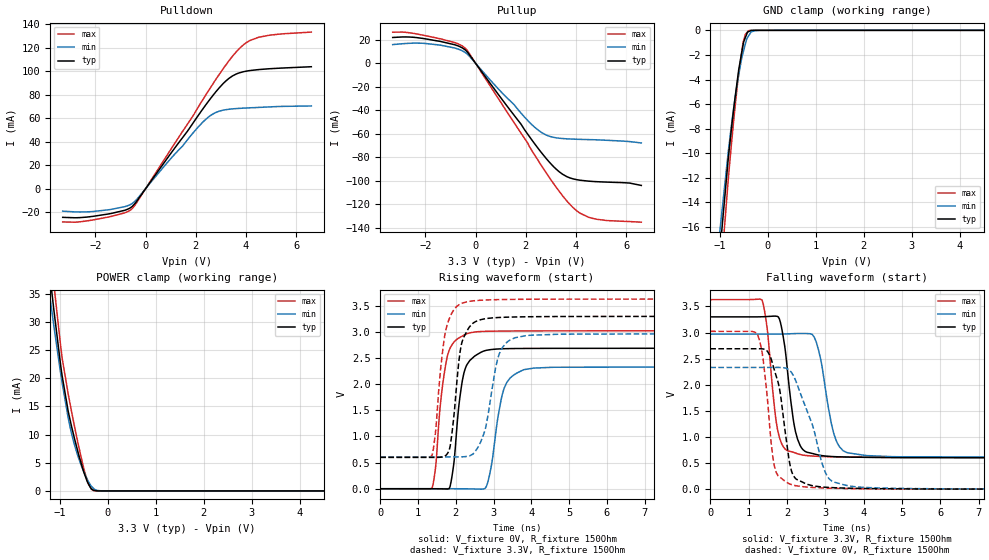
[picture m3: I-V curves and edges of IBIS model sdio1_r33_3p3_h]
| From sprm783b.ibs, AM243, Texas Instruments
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|   r33_3p3_h
[Model]   sdio1_r33_3p3_h
Model_type   I/O
Polarity   Non-Inverting
Enable   Active-High
Vinl = 0
Vinh = 0.8
Vmeas = 1.65
Vref = 3.3
Cref = 2pF
Rref = 100000
|   typ   min   max
C_comp   5.631pF   5.516pF   5.647pF
[Voltage Range]   3.3   2.97   3.63
[Temperature Range]   27   150   -40
[Pullup Reference]   3.3   2.97   3.63
[Pulldown Reference]   0   0   0
[Power Clamp Reference]   3.3   2.97   3.63
[GND Clamp Reference]   0   0   0
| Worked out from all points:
|   slope of the pulldown table from 0 to 0.495 V, typ, clamps not added: 33.3 ohm
|   slope of the pullup table from 0 to 0.495 V, typ, clamps not added: 34 ohm
|   GND clamp passes 1 mA (typ) near -0.51 V on its own axis
|   POWER clamp passes 1 mA (typ) near -0.39 V on its own axis
|   falling waveform, V_fixture 3.3V, R_fixture 150Ohm: 20-80 % time 275ps typ, 339ps min, 246ps max; typ from 3.3 V to 0.6 V
|   rising waveform, V_fixture 0V, R_fixture 150Ohm: 20-80 % time 240ps typ, 308ps min, 254ps max; typ from 0 V to 2.69 V
|   rising waveform, V_fixture 3.3V, R_fixture 150Ohm: 20-80 % time 238ps typ, 360ps min, 252ps max; typ from 0.6 V to 3.3 V
|   falling waveform, V_fixture 0V, R_fixture 150Ohm: 20-80 % time 336ps typ, 593ps min, 245ps max; typ from 2.69 V to 0 V
[Pulldown]
|   Voltage   I(typ)   I(min)   I(max)
-3.3V     -24.38mA   -19.12mA   -28.31mA
-2.102V   -23.55mA   -19.43mA   -26.62mA
-627mV    -16.54mA   -13.74mA   -18.54mA
-399.3mV  -12.02mA   -10.22mA   -13.37mA
838.2mV   25.12mA    21.55mA    27.93mA
2.363V    70.39mA    58.42mA    78.7mA
2.779V    82mA       64.74mA    92.43mA
3.175V    91.31mA    67.23mA    104.7mA
3.749V    98.78mA    68.44mA    119.7mA
4.125V    100.5mA    68.87mA    125.8mA
4.491V    101.4mA    69.21mA    128.9mA
6.6V      103.9mA    70.46mA    133.4mA
[GND Clamp]
|   Voltage   I(typ)   I(min)   I(max)
-3.3V     -160mA     -119.4mA   -217mA
-1.043V   -19.85mA   -17.9mA    -22.95mA
-825mV    -10.42mA   -9.877mA   -12.11mA
-696.3mV  -5.885mA   -5.888mA   -6.718mA
-607.2mV  -3.208mA   -3.602mA   -3.571mA
-528mV    -1.443mA   -2.001mA   -1.27mA
-508.2mV  -1.005mA   -1.701mA   -874.2uA
-468.6mV  -582.9uA   -1.101mA   -330.4uA
-399.3mV  -98.27uA   -431.3uA   -25.92uA
-349.8mV  -13.17uA   -132.1uA   -5.149uA
-171.6mV  -86.92nA   -2.806uA   -107.4nA
6.6V      0A         0A         0A
[Pullup]
|   Voltage   I(typ)   I(min)   I(max)
-3.3V     21.97mA    15.92mA    26.49mA
-2.468V   22.13mA    17.15mA    25.43mA
-1.449V   18.78mA    15.59mA    21.05mA
-825mV    15.76mA    12.98mA    17.59mA
-409.2mV  11.34mA    9.13mA     12.85mA
2.501V    -72.75mA   -57.03mA   -83.11mA
2.917V    -83.68mA   -61.97mA   -96.61mA
3.293V    -91.72mA   -63.71mA   -108mA
3.877V    -98.38mA   -64.58mA   -122.8mA
4.155V    -99.56mA   -64.79mA   -127.6mA
4.699V    -100.7mA   -65.1mA    -132.3mA
6.6V      -104mA     -67.83mA   -135.3mA
[POWER Clamp]
|   Voltage   I(typ)   I(min)   I(max)
-3.3V     224.5mA    191.3mA    262.6mA
-1.211V   38.57mA    34.7mA     44.22mA
-1.191V   37.06mA    33.44mA    42.47mA
-1.122V   31.9mA     29.08mA    36.46mA
-953.7mV  20.46mA    19.22mA    23.62mA
-825mV    14.07mA    12.89mA    17.14mA
-765.6mV  11.79mA    10.49mA    14.49mA
-636.9mV  7.377mA    6.549mA    9.056mA
-468.6mV  2.574mA    2.754mA    2.952mA
-399.3mV  1.162mA    1.587mA    1.17mA
-290.4mV  101.1uA    385.8uA    43.49uA
6.6V      0A         0A         0A
[Ramp]
R_load = 150
|   typ   min   max
dV/dt_r   1.61316/2.39024e-10   1.39818/3.0659e-10   1.81343/2.53741e-10
dV/dt_f   1.61988/2.74389e-10   1.41587/3.38839e-10   1.81501/2.45626e-10
[Falling Waveform]
V_fixture = 3.3V
V_fixture_min = 2.97V
V_fixture_max = 3.63V
R_fixture = 150Ohm
C_fixture = 0F
|   Time   V(typ)   V(min)   V(max)
0s        3.3V       2.969V     3.63V
1.35ns    3.302V     2.97V      3.621V
1.74ns    3.311V     2.97V      1.199V
2.015ns   2.254V     2.974V     736.5mV
2.185ns   1.239V     2.979V     702.4mV
2.375ns   795.7mV    2.982V     658.5mV
2.76ns    664.8mV    2.825V     630.8mV
3.21ns    624mV      1.093V     620.1mV
3.565ns   615.5mV    700mV      615.5mV
10ns      599.9mV    609.6mV    604.7mV
[Rising Waveform]
V_fixture = 0V
V_fixture_min = 0V
V_fixture_max = 0V
R_fixture = 150Ohm
C_fixture = 0F
|   Time   V(typ)   V(min)   V(max)
0s        356.1uV    864.9uV    228.3uV
1.37ns    221.6uV    569.7uV    13.01mV
1.63ns    -2.024mV   413.3uV    1.866V
1.825ns   6.295mV    450.6uV    2.651V
2.11ns    1.763V     -322.6uV   2.897V
2.285ns   2.361V     -1.532mV   2.963V
2.81ns    2.649V     46.35mV    3.013V
3.27ns    2.679V     1.903V     3.017V
3.795ns   2.684V     2.277V     3.02V
10ns      2.689V     2.331V     3.023V
[Rising Waveform]
V_fixture = 3.3V
V_fixture_min = 2.97V
V_fixture_max = 3.63V
R_fixture = 150Ohm
C_fixture = 0F
|   Time   V(typ)   V(min)   V(max)
0s        599.9mV    609.6mV    604.7mV
1.365ns   599.8mV    609.4mV    632.8mV
1.465ns   599.7mV    609.3mV    1.101V
1.675ns   613.9mV    609.2mV    2.772V
1.845ns   795.6mV    609.3mV    3.284V
2.16ns    2.796V     610.7mV    3.548V
2.66ns    3.235V     899.2mV    3.607V
3.145ns   3.277V     2.571V     3.619V
3.565ns   3.287V     2.889V     3.624V
10ns      3.3V       2.969V     3.63V
[Falling Waveform]
|Gnd
V_fixture = 0V
V_fixture_min = 0V
V_fixture_max = 0V
R_fixture = 150Ohm
C_fixture = 0F
|   Time   V(typ)   V(min)   V(max)
0s        2.689V     2.331V     3.023V
1.235ns   2.689V     2.331V     2.951V
1.38ns    2.685V     2.331V     2.474V
1.67ns    2.285V     2.331V     452mV
1.825ns   1.835V     2.331V     222mV
2.07ns    500mV      2.275V     100.1mV
2.235ns   195.5mV    2.065V     65.98mV
2.99ns    37.64mV    339.2mV    21.84mV
3.24ns    27.71mV    133.4mV    16.44mV
10ns      353.7uV    865uV      228.7uV
